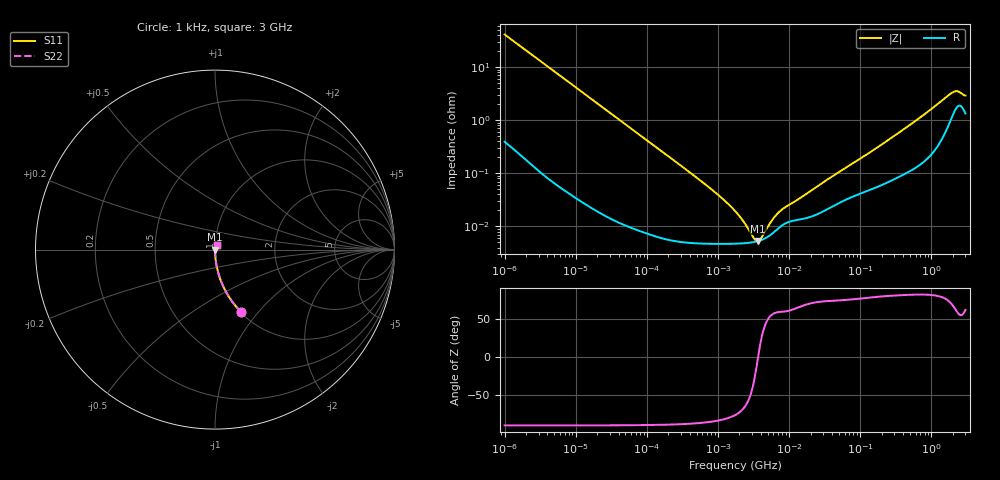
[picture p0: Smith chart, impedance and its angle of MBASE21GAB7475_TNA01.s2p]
! MBASE21GAB7475_TNA01  S-PARAMETER MODEL  ( Standard Model )
! Model Generated by TAIYO YUDEN Corporation (http://www.ty-top.com)
! Version 1.0
! TAIYO YUDEN Control No. 220601
! Copyright(c) 2012 TAIYO YUDEN CO.,LTD. All Rights Reserved.
! Product Description (link to TY-COMPAS)
! https://ds.yuden.co.jp/TYCOMPAS/or/detail?pn=MBASE21GAB7475KTNA01&u=M
! Products Name : Multilayer Ceramic Capacitors
! Characteristics :
!  Capacitance : 4.7 [uF] , Rated Voltage : 16 [V] , TCC : X7R
!  Case Size : 2.0 x 1.25 / 0.079 x 0.049 [mm/inch] , Thickness : 1.25 / 0.049 [mm/inch]
!  (Conditions: Temperature = 25 [degC] , DC Bias Voltage = 0 [V])
! External Node Assignments :
!  1  o---| |---o  2
! GND o---------o GND
! Frequency Range : 1kHz  -  3GHz  [ 401 STEP ]
# MHZ S RI R 50
! Freq[MHz].  S11 Real  S11 Imag  S21 Real  S21 Imag  S12 Real  S12 Imag  S22 Real  S22 Imag
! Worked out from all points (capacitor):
!   401 points, 1 kHz to 3 GHz, reference 50 ohm
!   read as one part in series: C = 3.86 uF near 1.077 kHz
!   lowest |Z| = 5.3 mohm at 3.651 MHz (marker M1)
!   series resonance near 3.653 MHz, so ESL is about 490 pH
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0.001  0.1469 -0.3492  0.8531 0.3492  0.8531 0.3492  0.1469 -0.3492
0.001685  0.0583 -0.23  0.9417 0.23  0.9417 0.23  0.0583 -0.23
0.003177  0.0177 -0.1278  0.9823 0.1278  0.9823 0.1278  0.0177 -0.1278
0.005768  0.0057 -0.0715  0.9943 0.0715  0.9943 0.0715  0.0057 -0.0715
0.01216  0.00146 -0.0342  0.9985 0.0342  0.9985 0.0342  0.00146 -0.0342
0.147855  7.01e-05 -0.00284  0.9999 0.00284  0.9999 0.00284  7.01e-05 -0.00284
0.791611  4.73e-05 -0.000509  1 0.000509  1 0.000509  4.73e-05 -0.000509
1.238299  4.7e-05 -0.000303  1 0.000303  1 0.000303  4.7e-05 -0.000303
1.732051  4.73e-05 -0.00019  1 0.00019  1 0.00019  4.73e-05 -0.00019
2.422679  4.85e-05 -9.88e-05  1 9.88e-05  1 9.88e-05  4.85e-05 -9.88e-05
2.610246  4.89e-05 -8.03e-05  1 8.03e-05  1 8.03e-05  4.89e-05 -8.03e-05
3.651041  5.3e-05 -1.4e-07  0.9999 1.4e-07  0.9999 1.4e-07  5.3e-05 -1.4e-07
4.919932  6.28e-05 7.13e-05  0.9999 -7.13e-05  0.9999 -7.13e-05  6.28e-05 7.13e-05
5.30084  6.71e-05 8.94e-05  0.9999 -8.94e-05  0.9999 -8.94e-05  6.71e-05 8.94e-05
6.629817  8.56e-05 0.000142  0.9999 -0.000142  0.9999 -0.000142  8.56e-05 0.000142
7.988506  0.000105 0.000181  0.9999 -0.000181  0.9999 -0.000181  0.000105 0.000181
21.06097  0.000156 0.000463  0.9998 -0.000463  0.9998 -0.000463  0.000156 0.000463
256.0921  0.000716 0.00432  0.9993 -0.00432  0.9993 -0.00432  0.000716 0.00432
700.8126  0.00159 0.0112  0.9984 -0.0112  0.9984 -0.0112  0.00159 0.0112
1917.819  0.0118 0.0299  0.9882 -0.0299  0.9882 -0.0299  0.0118 0.0299
2310.849  0.0184 0.0291  0.9816 -0.0291  0.9816 -0.0291  0.0184 0.0291
3000  0.0139 0.025  0.9861 -0.025  0.9861 -0.025  0.0139 0.025
